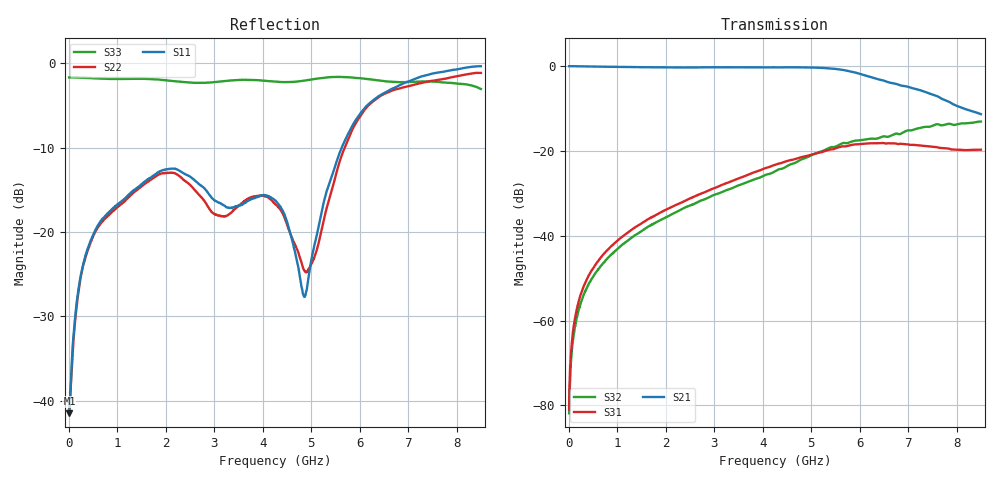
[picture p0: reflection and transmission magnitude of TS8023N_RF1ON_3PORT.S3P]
!Agilent Technologies,E5071C,MY46522130,B.12.04
!Date: Thu Jul 17 20:35:12 2025
!Data & Calibration Information:
!Freq	S11:SOLT3(ON)	S13:SOLT3(ON)	S14:SOLT3(ON)
!	S31:SOLT3(ON)	S33:SOLT3(ON)	S34:SOLT3(ON)
!	S41:SOLT3(ON)	S43:SOLT3(ON)	S44:SOLT3(ON)
!PortZ  Port1:50+j0  Port3:50+j0  Port4:50+j0
!Above PortZ is port z conversion or system Z0 setting when saving the data.
!When reading, reference impedance value at option line is always used.
# Hz S dB R 50
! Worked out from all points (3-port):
!   1601 points, 10 MHz to 8.5 GHz, reference 50 ohm
!   strongest paths, dB at 10 MHz, 2.132 GHz, 4.255 GHz, 6.378 GHz, 8.5 GHz:
!     S21: -0.1, -0.4, -0.4, -3.2, -11.4
!     S31: -80.9, -33.2, -23.4, -18.3, -19.8
!     S32: -81.9, -35.0, -24.9, -17.1, -13.2
!   lowest |S11| = -41.5 dB at 15.31 MHz (marker M1), VSWR 1.02, Z = 50.8 - j0.276 ohm
!   |S11| at or under -10 dB: start of sweep to 5.631 GHz
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1e7  -41.21 -9.5  -0.12 -0.2  -80.88 53.7
     -0.11 -0.2  -41.01 -7.9  -81.16 48.6
     -80.93 62.7  -81.85 50.5  -1.70 179.8
1.530625e7  -41.49 -18.8  -0.12 -0.4  -76.56 69.8
            -0.11 -0.3  -40.99 -16.9  -78.03 73.1
            -76.77 71.6  -78.29 61.7  -1.69 179.8
2.063312e8  -26.66 -85.2  -0.14 -4.3  -55.48 87.9
            -0.14 -4.4  -26.88 -88.0  -57.53 87.5
            -55.56 88.4  -57.57 87.5  -1.72 177.8
7.475688e8  -18.14 -97.0  -0.24 -15.2  -44.02 91.2
            -0.24 -15.2  -18.42 -107.3  -46.00 90.3
            -44.05 91.1  -46.06 90.2  -1.85 169.6
2.09005e9  -12.53 -111.8  -0.43 -41.3  -33.46 86.9
           -0.43 -41.3  -12.98 -144.2  -35.15 84.7
           -33.46 86.9  -35.21 84.8  -2.08 145.0
4.255e9  -16.24 -121.9  -0.42 -88.2  -23.48 57.7
         -0.40 -88.3  -16.70 129.8  -24.96 61.7
         -23.35 57.9  -24.88 61.9  -2.18 97.6
4.865219e9  -27.68 161.0  -0.40 -104.4  -21.41 42.7
            -0.40 -104.5  -24.60 155.3  -21.85 50.9
            -21.34 42.7  -21.79 51.0  -2.07 81.7
6.043206e9  -5.75 100.0  -1.99 -144.8  -18.40 6.2
            -2.03 -145.0  -6.00 142.0  -17.58 15.1
            -18.42 6.4  -17.51 15.8  -1.80 77.3
7.26895e9  -1.58 54.0  -5.91 -174.3  -18.80 -28.1
           -5.83 -174.5  -2.35 130.0  -14.45 -15.7
           -18.82 -28.3  -14.60 -16.1  -2.18 59.5
8.5e9  -0.37 57.0  -11.29 174.3  -19.78 -44.7
       -11.40 174.7  -1.16 99.6  -13.28 -41.5
       -19.78 -44.3  -13.15 -41.5  -3.06 56.4
